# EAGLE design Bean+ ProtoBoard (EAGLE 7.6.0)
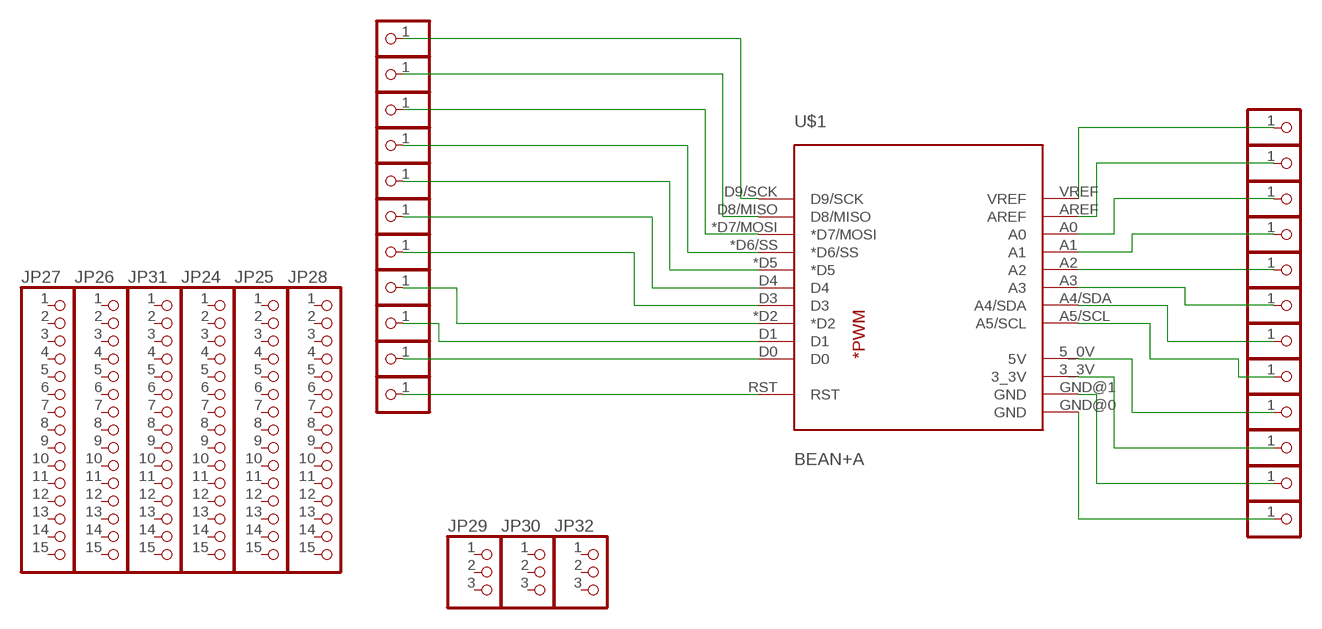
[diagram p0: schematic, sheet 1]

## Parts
JP1  PINHD-1X1CB  [1X01-CLEANBIG]
JP2  PINHD-1X1CB  [1X01-CLEANBIG]
JP3  PINHD-1X1CB  [1X01-CLEANBIG]
JP4  PINHD-1X1CB  [1X01-CLEANBIG]
JP5  PINHD-1X1CB  [1X01-CLEANBIG]
JP6  PINHD-1X1CB  [1X01-CLEANBIG]
JP7  PINHD-1X1CB  [1X01-CLEANBIG]
JP8  PINHD-1X1CB  [1X01-CLEANBIG]
JP9  PINHD-1X1CB  [1X01-CLEANBIG]
JP10  PINHD-1X1CB  [1X01-CLEANBIG]
JP11  PINHD-1X1CB  [1X01-CLEANBIG]
JP12  PINHD-1X1CB  [1X01-CLEANBIG]
JP13  PINHD-1X1CB  [1X01-CLEANBIG]
JP14  PINHD-1X1CB  [1X01-CLEANBIG]
JP15  PINHD-1X1CB  [1X01-CLEANBIG]
JP16  PINHD-1X1CB  [1X01-CLEANBIG]
JP17  PINHD-1X1CB  [1X01-CLEANBIG]
JP18  PINHD-1X1CB  [1X01-CLEANBIG]
JP19  PINHD-1X1CB  [1X01-CLEANBIG]
JP20  PINHD-1X1CB  [1X01-CLEANBIG]
JP21  PINHD-1X1CB  [1X01-CLEANBIG]
JP22  PINHD-1X1CB  [1X01-CLEANBIG]
JP23  PINHD-1X1CB  [1X01-CLEANBIG]
JP24  PINHD-1X15-CB  [1X15-CB]
JP25  PINHD-1X15-CB  [1X15-CB]
JP26  PINHD-1X15-CB  [1X15-CB]
JP27  PINHD-1X15-CB  [1X15-CB]
JP28  PINHD-1X15-CB  [1X15-CB]
JP29  PINHD-1X3  [1X03]
JP30  PINHD-1X3  [1X03]
JP31  PINHD-1X15-CB  [1X15-CB]
JP32  PINHD-1X3  [1X03]
U$1  BEAN+A  [BEAN+]

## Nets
N$1: JP22.1 U$1.*D7/MOSI
N$2: JP23.1 U$1.D8/MISO
N$3: JP3.1 U$1.*D6/SS
N$4: JP4.1 U$1.*D5
N$5: JP5.1 U$1.D4
N$6: JP6.1 U$1.D3
N$7: JP7.1 U$1.*D2
N$8: JP8.1 U$1.D1
N$9: JP9.1 U$1.D0
N$10: JP10.1 U$1.RST
N$11: JP11.1 U$1.VREF
N$12: JP12.1 U$1.AREF
N$13: JP13.1 U$1.A0
N$14: JP14.1 U$1.A1
N$15: JP15.1 U$1.A2
N$16: JP16.1 U$1.A3
N$17: JP21.1 U$1.GND@1(GND)
N$18: JP17.1 U$1.A4/SDA
N$19: JP18.1 U$1.A5/SCL
N$20: JP19.1 U$1.5_0V(5V)
N$21: JP20.1 U$1.3_3V
N$22: JP1.1 U$1.D9/SCK
N$23: JP2.1 U$1.GND@0(GND)
Unconnected: JP24.1 JP24.2 JP24.3 JP24.4 JP24.5 JP24.6 JP24.7 JP24.8 JP24.9 JP24.10 JP24.11 JP24.12 JP24.13 JP24.14 JP24.15 JP25.1 JP25.2 JP25.3 JP25.4 JP25.5 JP25.6 JP25.7 JP25.8 JP25.9 JP25.10 JP25.11 JP25.12 JP25.13 JP25.14 JP25.15 JP26.1 JP26.2 JP26.3 JP26.4 JP26.5 JP26.6 JP26.7 JP26.8 JP26.9 JP26.10 JP26.11 JP26.12 JP26.13 JP26.14 JP26.15 JP27.1 JP27.2 JP27.3 JP27.4 JP27.5 JP27.6 JP27.7 JP27.8 JP27.9 JP27.10 JP27.11 JP27.12 JP27.13 JP27.14 JP27.15 JP28.1 JP28.2 JP28.3 JP28.4 JP28.5 JP28.6 JP28.7 JP28.8 JP28.9 JP28.10 JP28.11 JP28.12 JP28.13 JP28.14 JP28.15 JP29.1 JP29.2 JP29.3 JP30.1 JP30.2 JP30.3 JP31.1 JP31.2 JP31.3 JP31.4 JP31.5 JP31.6 JP31.7 JP31.8 JP31.9 JP31.10 JP31.11 JP31.12 JP31.13 JP31.14 JP31.15 JP32.1 JP32.2 JP32.3

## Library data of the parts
JP1-JP23 = adafruit:PINHD-1X1: Pin header 1x1 for 0.1" spacing
JP24-JP28 JP31 = adafruit:PINHD-1X15: PIN HEADER
JP29 JP30 JP32 = adafruit:PINHD-1X3: PIN HEADER
U$1 = Bean+:BEAN+: Bean+ Shield

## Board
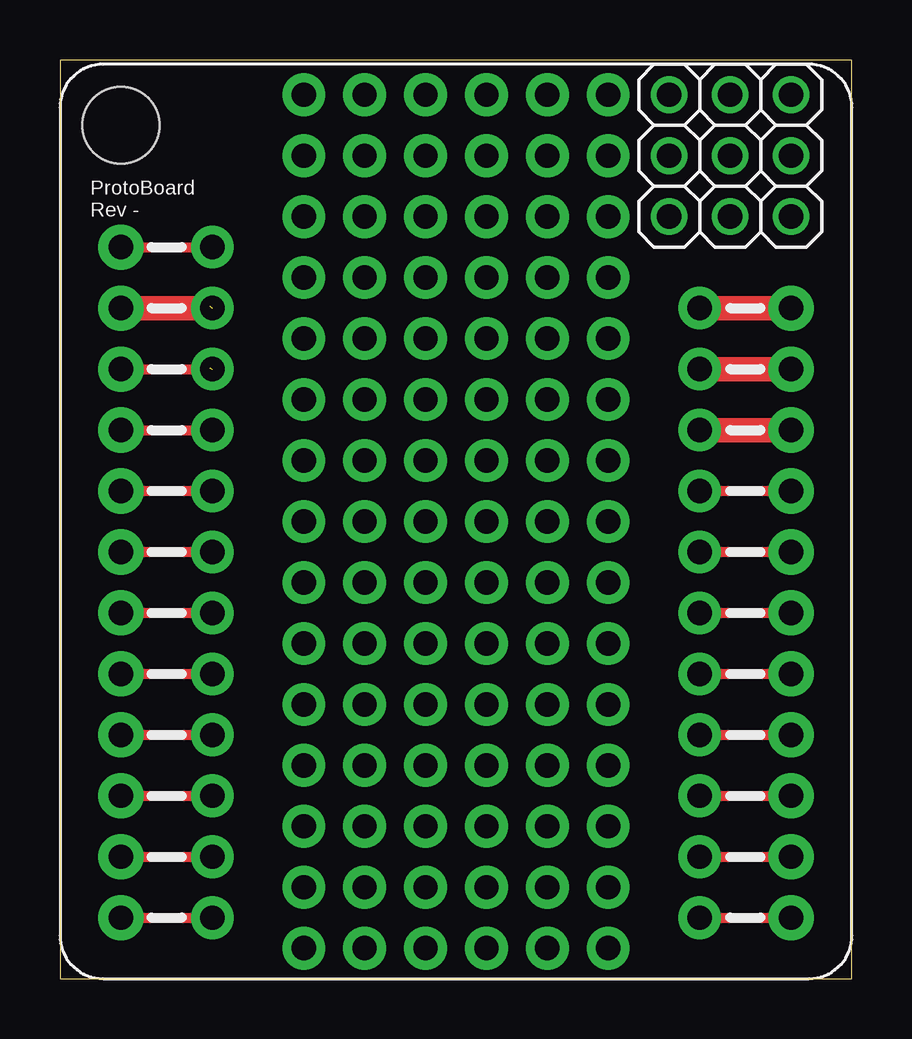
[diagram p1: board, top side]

Size 33 x 38.28 mm. Coordinates in mm from the lower left corner, seen from the top.
Outline: 0,0 33,0 33,38.28 0,38.28 0,0
Copper layers (1*16): Top 0.0356mm / dielectric 1.5011mm / Bottom 0.0356mm
Design rules "oshpark-2layer": minimum track width 6mil, minimum drill 13mil, track to track 6mil, track to pad 6mil, pad to pad 6mil, via to via 6mil, smd to smd 6mil, copper to edge 15mil, drill to drill 6mil, minimum pad ring 7mil, minimum via ring 7mil, stop-mask expansion 2.5mil, vias tented up to drill 0mil, thermal gap 10mil

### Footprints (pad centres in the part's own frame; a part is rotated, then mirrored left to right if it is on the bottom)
1X01-CLEANBIG = drill 1.016 pad 1.778: 1 0,0
1X15-CB = drill 1.016 pad 1.778: 1 -17.78,0; 2 -15.24,0; 3 -12.7,0; 4 -10.16,0; 5 -7.62,0; 6 -5.08,0; 7 -2.54,0; 8 0,0; 9 2.54,0; 10 5.08,0; 11 7.62,0; 12 10.16,0; 13 12.7,0; 14 15.24,0; 15 17.78,0
1X03 = drill 1.016: 1 -2.54,0; 2 0,0; 3 2.54,0
BEAN+ = drill 1.016 pad 1.88: 3_3V 13.97,6.35; 5_0V 13.97,3.81; *D2 -13.97,-11.43; *D5 -13.97,-3.81; *D6/SS -13.97,-1.27; *D7/MOSI -13.97,1.27; A0 13.97,-3.81; A1 13.97,-6.35; A2 13.97,-8.89; A3 13.97,-11.43; A4/SDA 13.97,-13.97; A5/SCL 13.97,-16.51; AREF 13.97,-1.27; D0 -13.97,-16.51; D1 -13.97,-13.97; D3 -13.97,-8.89; D4 -13.97,-6.35; D8/MISO -13.97,3.81; D9/SCK -13.97,6.35; GND@0 -13.97,8.89; GND@1 13.97,8.89; RST -13.97,11.43; VREF 13.97,1.27 | hole 3.2: -13.97,16.51

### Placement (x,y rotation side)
JP1  6.35,25.4 0 top
JP2  6.35,27.94 0 top
JP3  6.35,17.78 0 top
JP4  6.35,15.24 0 top
JP5  6.35,12.7 0 top
JP6  6.35,10.16 0 top
JP7  6.35,7.62 0 top
JP8  6.35,5.08 0 top
JP9  6.35,2.54 0 top
JP10  6.35,30.48 0 top
JP11  26.67,20.32 0 top
JP12  26.67,17.78 0 top
JP13  26.67,15.24 0 top
JP14  26.67,12.7 0 top
JP15  26.67,10.16 0 top
JP16  26.67,7.62 0 top
JP17  26.67,5.08 0 top
JP18  26.67,2.54 0 top
JP19  26.67,22.86 0 top
JP20  26.67,25.4 0 top
JP21  26.67,27.94 0 top
JP22  6.35,20.32 0 top
JP23  6.35,22.86 0 top
JP24  12.7,19.05 90 top
JP25  15.24,19.05 90 top
JP26  17.78,19.05 90 top
JP27  20.32,19.05 90 top
JP28  22.86,19.05 90 top
JP29  25.4,34.29 90 top
JP30  27.94,34.29 90 top
JP31  10.16,19.05 90 top
JP32  30.48,34.29 90 top
U$1  16.51,19.05 0 top

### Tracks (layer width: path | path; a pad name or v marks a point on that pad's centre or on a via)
N$1
  Top 0.406: U$1.*D7/MOSI JP22.1
N$2
  Top 0.406: U$1.D8/MISO JP23.1
N$3
  Top 0.406: U$1.*D6/SS JP3.1
N$4
  Top 0.406: U$1.*D5 JP4.1
N$5
  Top 0.406: U$1.D4 JP5.1
N$6
  Top 0.406: U$1.D3 JP6.1
N$7
  Top 0.406: U$1.*D2 JP7.1
N$8
  Top 0.406: U$1.D1 JP8.1
N$9
  Top 0.406: U$1.D0 JP9.1
N$10
  Top 0.406: U$1.RST JP10.1
N$11
  Top 0.406: JP11.1 U$1.VREF
N$12
  Top 0.406: JP12.1 U$1.AREF
N$13
  Top 0.406: JP13.1 U$1.A0
N$14
  Top 0.406: JP14.1 U$1.A1
N$15
  Top 0.406: JP15.1 U$1.A2
N$16
  Top 0.406: JP16.1 U$1.A3
N$17
  Top 1.016: JP21.1 U$1.GND@1
N$18
  Top 0.406: JP17.1 U$1.A4/SDA
N$19
  Top 0.406: JP18.1 U$1.A5/SCL
N$20
  Top 1.016: JP19.1 U$1.5_0V
N$21
  Top 1.016: JP20.1 U$1.3_3V
N$22  (1 unrouted)
  Top 0.406: U$1.D9/SCK JP1.1
N$23  (1 unrouted)
  Top 1.016: U$1.GND@0 JP2.1

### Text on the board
tNames: ProtoBoard / Rev -
bNames: ProtoBoard / Rev -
